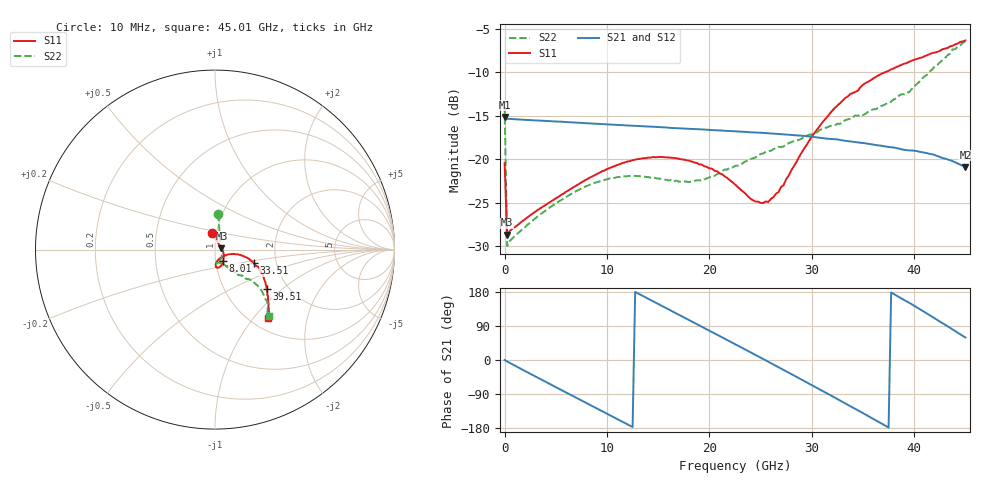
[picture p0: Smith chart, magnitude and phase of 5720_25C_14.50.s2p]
! Device:  ADRF5720
! Description: 0.5dB LSB GaAs MMIC 6-bit Digital Attenuator
! Frequency:  0.000009 -  40 GHz
! Ports:
!	RF1	= Port 1
!	RF2	= Port 2
! Vdd:  3.3 Volt
! Vss:  -3.3 Volt
! Control:  0/3.3 Volt
! State:  14.50 dB attenuation
! Data:  The device was measured using G-S-G Probes on a matrix board.
!  Data was collected using an calibrated 4 port network analyzer.
!  The reference plane for this measurement is at the launchers.
! Note:  Analog Devices supplies this data as a sample of measured data
!  for this product.  Your particular data for this product may vary.
!  Data was taken at 25 degrees C.
!  Analog Devices reserves the right to change this data at anytime.
# GHZ S DB R 45.0
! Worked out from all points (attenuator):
!   181 points, 10 MHz to 45.01 GHz, reference 45 ohm
!   highest |S21| = -15.16 dB at 10 MHz (marker M1); lowest = -20.9 dB at 45.01 GHz (marker M2)
!   lowest |S11| = -28.7 dB at 260 MHz (marker M3), VSWR 1.08, Z = 48.3 + j0.802 ohm
!   |S11| at or under -10 dB: start of sweep to 37.16 GHz
!   |S22| runs from -30.0 to -6.4 dB; largest |S21 - S12| = 0.00023
!   S11 on the Smith chart (normalised r, x): 10 MHz: 0.95, +0.18; 8.01 GHz: 1.09, -0.13; 33.51 GHz: 1.53, -0.24; 39.51 GHz: 1.56, -0.80; 45.01 GHz: 1.19, -1.19
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0.01  -20.49 100.2  -15.16 -0.1  -15.16 -0.1  -14.01 84.7
0.26  -28.70 13.0  -15.35 -4.0  -15.36 -4.0  -30.03 14.0
1.26  -27.62 -2.9  -15.42 -18.5  -15.43 -18.5  -28.59 -7.3
4.26  -25.08 -30.3  -15.61 -61.0  -15.62 -61.0  -25.71 -42.8
7.76  -22.51 -51.4  -15.84 -110.3  -15.84 -110.3  -23.24 -66.3
8.01  -22.34 -52.7  -15.86 -113.8  -15.86 -113.8  -23.10 -67.5
11.76  -20.37 -69.0  -16.11 -166.3  -16.11 -166.3  -21.98 -81.0
15.26  -19.75 -80.5  -16.32 144.3  -16.32 144.4  -22.27 -84.5
19.01  -20.60 -87.3  -16.56 91.5  -16.57 91.5  -22.43 -72.3
21.26  -21.75 -86.7  -16.71 59.6  -16.72 59.6  -21.36 -64.5
22.76  -23.20 -82.4  -16.81 38.3  -16.82 38.4  -20.76 -60.2
24.26  -24.74 -69.0  -16.92 17.0  -16.93 17.0  -19.92 -57.4
25.76  -24.92 -45.3  -17.02 -4.6  -17.02 -4.5  -19.07 -55.7
27.26  -22.99 -24.0  -17.14 -26.3  -17.14 -26.3  -18.54 -53.2
30.26  -17.01 -11.8  -17.46 -70.0  -17.47 -70.0  -16.97 -51.1
32.01  -14.41 -14.7  -17.70 -95.6  -17.70 -95.5  -16.15 -50.2
33.51  -12.79 -19.3  -17.92 -117.9  -17.93 -117.9  -15.42 -48.6
35.51  -11.09 -25.1  -18.23 -147.9  -18.23 -147.9  -14.55 -47.0
37.76  -9.65 -32.4  -18.63 178.1  -18.63 178.2  -13.38 -43.4
39.51  -8.79 -37.5  -19.00 151.2  -19.00 151.2  -12.29 -42.2
42.26  -7.65 -44.4  -19.63 105.5  -19.63 105.6  -9.16 -41.5
45.01  -6.33 -52.5  -20.90 59.4  -20.91 59.5  -6.42 -51.0
